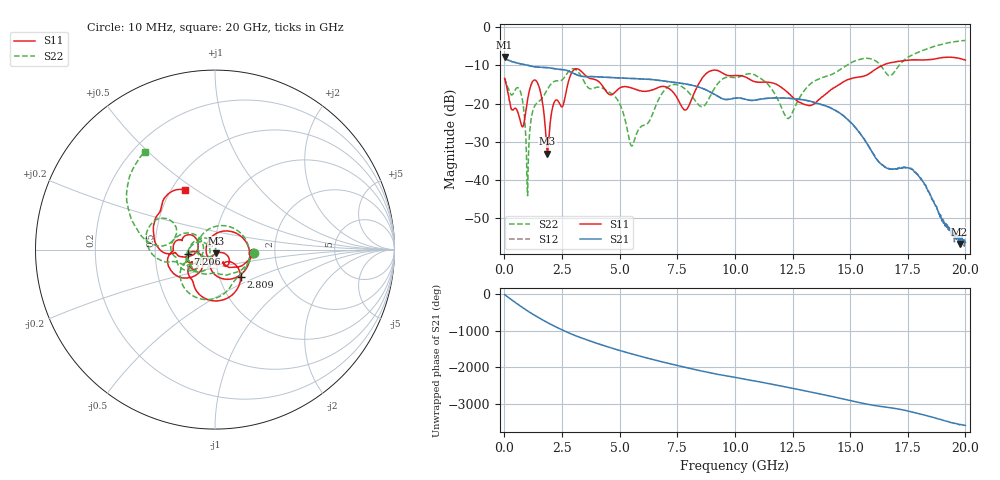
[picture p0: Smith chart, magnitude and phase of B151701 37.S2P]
!  2-Port S-parameters saved by WinCal
! VAR MeasName=S-Parameters (CALIBRATED_DATA) read from VNA (N5244A)
! VAR MeasDate=2015-12-24 19:13:41
! VAR NAME=B151701 37
! VAR FILENAME=B151701 37.S2P
! VAR DATE=2015-12-24 19:13:41
! VAR PHYS_PORTS=1,3
# Hz S DB R 50
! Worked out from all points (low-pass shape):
!   801 points, 10 MHz to 20 GHz, reference 50 ohm
!   highest |S21| = -7.77 dB at 10 MHz (marker M1); lowest = -56.7 dB at 19.75 GHz (marker M2)
!   |S21| within 3 dB of the highest: start of sweep to 2.082 GHz
!   lowest |S11| = -33.1 dB at 1.859 GHz (marker M3), VSWR 1.05, Z = 50.5 - j2.16 ohm
!   |S11| at or under -10 dB: start of sweep to 16.39 GHz
!   |S22| runs from -44.1 to -3.5 dB; largest |S21 - S12| = 0.0012
!   S11 on the Smith chart (normalised r, x): 10 MHz: 1.54, -0.06; 2.809 GHz: 1.26, -0.40; 7.206 GHz: 0.74, -0.04; 20 GHz: 0.59, +0.45
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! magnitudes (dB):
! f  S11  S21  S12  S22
! 10 MHz  -13.4  -7.8  -7.8  -13.3
! 709.6 MHz  -25.0  -9.6  -9.6  -17.1
! 1.01 GHz  -18.9  -9.9  -9.9  -44.1
! 1.434 GHz  -14.5  -10.5  -10.4  -19.7
! 1.859 GHz  -33.1  -10.6  -10.6  -16.4
! 2.809 GHz  -13.6  -11.5  -11.5  -11.4
! 3.358 GHz  -11.7  -12.8  -12.8  -13.1
! 4.858 GHz  -16.6  -13.2  -13.2  -18.6
! 5.532 GHz  -15.9  -13.4  -13.4  -31.1
! 6.682 GHz  -15.8  -13.9  -13.9  -19.0
! 7.206 GHz  -16.4  -14.3  -14.4  -15.2
! 7.856 GHz  -21.6  -14.8  -14.9  -16.2
! 8.581 GHz  -13.3  -16.0  -16.0  -20.8
! 10.01 GHz  -12.6  -18.6  -18.5  -13.2
! 11.23 GHz  -14.4  -18.7  -18.7  -13.9
! 12.3 GHz  -17.1  -18.6  -18.6  -23.9
! 13.35 GHz  -20.3  -19.5  -19.5  -14.5
! 15.63 GHz  -12.7  -29.4  -29.4  -8.2
! 16.68 GHz  -9.4  -37.1  -37.0  -12.6
! 17.83 GHz  -8.5  -38.0  -37.9  -6.9
! 19.75 GHz  -8.2  -56.7  -55.9  -3.6
! 20 GHz  -8.6  -56.3  -56.2  -3.5
